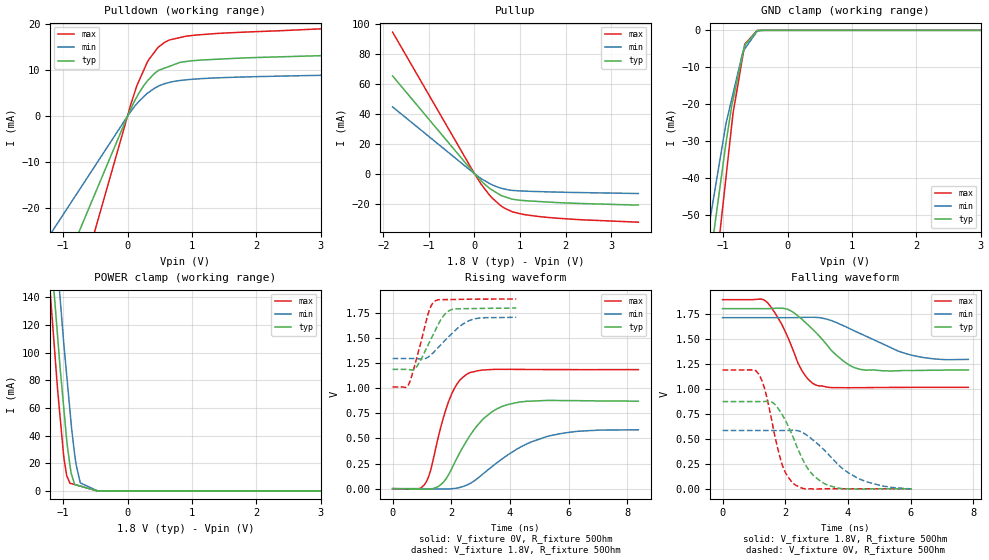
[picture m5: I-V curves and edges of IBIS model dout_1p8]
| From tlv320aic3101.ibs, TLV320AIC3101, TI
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|   dout_1p8 Model
[Model]   dout_1p8
Model_type   3-state
Polarity   Non-Inverting
Vmeas = 0.9
Vref = 0.9
Cref = 10pF
Rref = 50
|   typ   min   max
|   (nom PVT)   (fast PVT)   (slow PVT)
 C_comp   1.417e-12   1.397e-12   1.458e-12
| Where nom  PVT is Nominal Process, 1.8V, 27C
|   Fast PVT is Strong Process,  1.89V, -40C
|   Slow PVT is Weak Process,   1.71V, 105C
[Voltage Range]   1.8   1.71   1.89
|Ambient Temperature   25   85   -40
|Junction Temperature
[Temperature Range]   27   105   -40
[Pullup Reference]   1.8   1.71   1.89
[Pulldown Reference]   0   0   0
[Power Clamp Reference]   1.8   1.71   1.89
[GND Clamp Reference]   0   0   0
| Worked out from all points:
|   slope of the pulldown table from 0 to 0.27 V, typ, clamps not added: 38.8 ohm
|   slope of the pullup table from 0 to 0.27 V, typ, clamps not added: 32.8 ohm
|   GND clamp passes 1 mA (typ) near -0.52 V on its own axis
|   falling waveform, V_fixture 1.8V, R_fixture 50Ohm: 20-80 % time 1.14ns typ, 1.72ns min, 762ps max; typ from 1.8 V to 1.19 V
|   rising waveform, V_fixture 0V, R_fixture 50Ohm: 20-80 % time 1.13ns typ, 1.8ns min, 682ps max; typ from 0 V to 0.872 V
|   rising waveform, V_fixture 1.8V, R_fixture 50Ohm: 20-80 % time 622ps typ, 866ps min, 466ps max; typ from 1.19 V to 1.8 V
|   falling waveform, V_fixture 0V, R_fixture 50Ohm: 20-80 % time 804ps typ, 1.29ns min, 521ps max; typ from 0.871 V to 0 V
[Pulldown]
|   Voltage   I(typ)   I(min)   I(max)
-1.8V     -59.89mA   -38.41mA   -88.18mA
-66.6mV   -2.216mA   -1.421mA   -3.263mA
51.03mV   1.569mA    1.01mA     2.575mA
145.5mV   4.212mA    2.715mA    6.623mA
252mV     6.622mA    4.23mA     9.986mA
302.4mV   7.55mA     4.897mA    11.57mA
470.6mV   9.821mA    6.44mA     14.86mA
574.6mV   10.42mA    7.046mA    16mA
655.8mV   10.84mA    7.342mA    16.54mA
817.2mV   11.67mA    7.747mA    17.05mA
1.139V    12.17mA    8.129mA    17.67mA
3.6V      13.41mA    9.027mA    19.33mA
[GND Clamp]
|   Voltage   I(typ)   I(min)   I(max)
-1.8V     -212.8mA   -128.2mA   -311.2mA
-1.411V   -94.16mA   -73.15mA   -120.3mA
-1.147V   -55.07mA   -45.31mA   -70.45mA
-1.138V   -53.93mA   -44.38mA   -68.79mA
-959.3mV  -30.92mA   -25.56mA   -40.39mA
-867.6mV  -20.6mA    -18.72mA   -25.8mA
-846.7mV  -18.85mA   -17.17mA   -22.52mA
-692.5mV  -6.238mA   -5.727mA   -6.74mA
-663.4mV  -4.012mA   -5.002mA   -3.754mA
-470.6mV  -77.09uA   -204.9uA   -26.21uA
-289mV    -483.8nA   -2.468uA   -108.9nA
3.6V      0A         0A         0A
[Pullup]
|   Voltage   I(typ)   I(min)   I(max)
-1.8V     65.23mA    44.56mA    94.44mA
0V        0A         0A         0A
151.2mV   -4.943mA   -3.327mA   -7.217mA
332.6mV   -9.769mA   -6.557mA   -14.34mA
574.6mV   -14.37mA   -9.577mA   -21.25mA
835.4mV   -16.98mA   -11.14mA   -25.46mA
1.058V    -17.83mA   -11.55mA   -27.07mA
1.382V    -18.48mA   -11.9mA    -28.45mA
2.268V    -19.79mA   -12.55mA   -30.57mA
3.6V      -20.92mA   -13.2mA    -32.33mA
[POWER Clamp]
|   Voltage   I(typ)   I(min)   I(max)
-1.8V     564.6mA    604.4mA    540.6mA
-1.219V   190.5mA    240.9mA    154.2mA
-1.161V   155.5mA    205mA      119mA
-1.087V   112mA      162.1mA    73.48mA
-1.049V   90.18mA    140.6mA    54.51mA
-988.5mV  59.01mA    105.5mA    23.98mA
-945mV    36.78mA    83.62mA    11.02mA
-894mV    18.49mA    57.87mA    5.566mA
-820.8mV  4.604mA    26.11mA    4.609mA
-733.6mV  3.471mA    5.818mA    3.468mA
-470.3mV  64.54uA    115.8uA    28.17uA
3.6V      0A         0A         0A
[Ramp]
R_load = 50
|   typ   min   max
dV/dt_r   0.522874/1.12249e-09   0.349429/1.76973e-09   0.712031/6.78747e-10
dV/dt_f   0.366677/1.12938e-09   0.247668/1.70322e-09   0.525797/7.60521e-10
[Falling Waveform]
V_fixture = 1.8V
V_fixture_min = 1.71V
V_fixture_max = 1.89V
R_fixture = 50Ohm
|   Time   V(typ)   V(min)   V(max)
0s        1.8V       1.71V      1.89V
1.408ns   1.8V       1.71V      1.868V
1.876ns   1.805V     1.71V      1.651V
2.146ns   1.783V     1.71V      1.467V
2.54ns    1.692V     1.713V     1.177V
2.972ns   1.564V     1.713V     1.037V
3.834ns   1.282V     1.633V     1.01V
4.386ns   1.193V     1.552V     1.011V
6.032ns   1.182V     1.335V     1.013V
7.842ns   1.187V     1.293V     1.014V
[Rising Waveform]
V_fixture = 0V
V_fixture_min = 0V
V_fixture_max = 0V
R_fixture = 50Ohm
|   Time   V(typ)   V(min)   V(max)
0s        1.155nV    20.9nV     619.9pV
1.09ns    -5.181mV   -512.7uV   41.25mV
1.302ns   -3.153mV   -3.02mV    189mV
1.58ns    26.23mV    -4.186mV   539.7mV
1.99ns    184mV      -1.629mV   928.1mV
2.612ns   518mV      47.33mV    1.153V
3.378ns   764.1mV    217.3mV    1.188V
4.222ns   857.4mV    391.5mV    1.189V
5.816ns   877.8mV    553.4mV    1.187V
8.374ns   872mV      587mV      1.187V
[Rising Waveform]
V_fixture = 1.8V
V_fixture_min = 1.71V
V_fixture_max = 1.89V
R_fixture = 50Ohm
|   Time   V(typ)   V(min)   V(max)
0s        1.189V     1.297V     1.014V
548ps     1.188V     1.297V     1.038V
820ps     1.214V     1.297V     1.299V
1.208ns   1.431V     1.311V     1.741V
1.324ns   1.5V       1.338V     1.828V
1.462ns   1.582V     1.378V     1.874V
1.772ns   1.736V     1.473V     1.885V
2.022ns   1.786V     1.546V     1.885V
2.754ns   1.795V     1.691V     1.889V
4.214ns   1.8V       1.709V     1.89V
[Falling Waveform]
V_fixture = 0V
V_fixture_min = 0V
V_fixture_max = 0V
R_fixture = 50Ohm
|   Time   V(typ)   V(min)   V(max)
0s        871.5mV    582.4mV    1.187V
1.14ns    871.4mV    582.4mV    1.152V
1.378ns   872.9mV    582.4mV    958.3mV
1.626ns   855.4mV    582.4mV    592.6mV
1.872ns   755.9mV    582.3mV    268.7mV
2.334ns   451.1mV    583.4mV    35.79mV
2.808ns   164.5mV    507.8mV    377.1uV
3.37ns    35.5mV     346.1mV    622.6uV
4.434ns   -3.692mV   89.07mV    -41.96uV
6.038ns   -33.65uV   -1.654mV   -36.22uV
